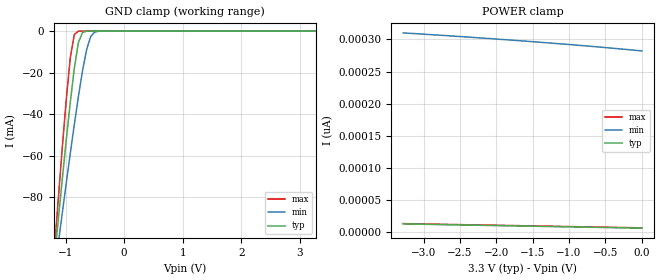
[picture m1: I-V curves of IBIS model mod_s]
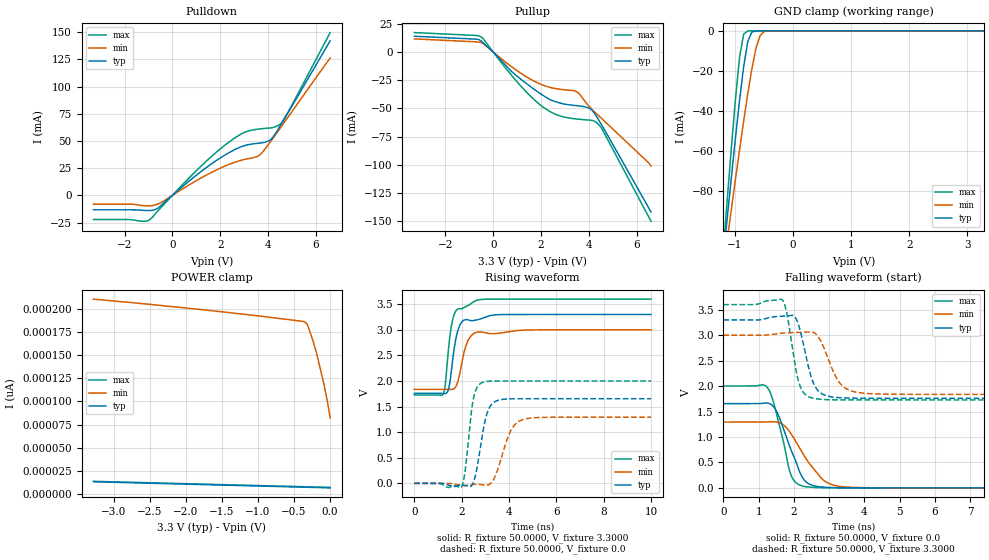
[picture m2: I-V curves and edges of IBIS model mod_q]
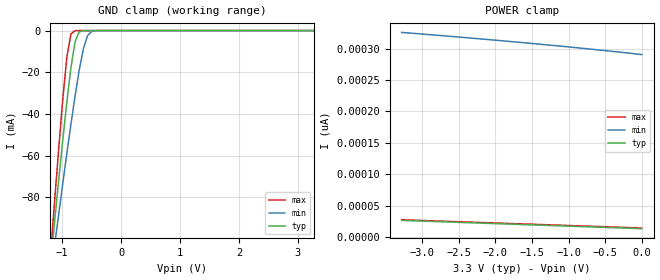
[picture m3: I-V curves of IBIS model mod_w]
| IBIS (I/O, Buffer, Information, Specification) Model, officially
| electronic behavioral standard for Buffer structures of digital pins.
[IBIS ver]  4.0
[File name] m95m02e-a125_3v3_tssop08.ibs
[File Rev]  1.0
[Date]   12 March 2025
[Source]   CAD & Design Services (Catania) - STMicroelectronics
[Notes]
   (Note1)  This IBIS model includes TSSOP8 Package parasitic data
   (Note2)  This IBIS model considers: VCC=3.30(TYP), 3.00(MIN), 3.60(MAX)
   (Note3)  This IBIS model has some Notes about the non-monotonicity
   of the I-V curves, but they are not indicative of problems
   inside the model;
[Disclaimer]
   Customers are solely responsible for all aspects of their
   own product designs or applications using this IBIS Model.
   STMicroelectronics assumes no liability for Custmer Designs
   and applications associated to this IBIS Model.
   In the use of this IBIS Model Customer shall not modify,
   disassemble, alter this Model in whole or in part.
   If Customers do not accept these terms, the IBIS Model
   may not be used. For any problems or modifications please
   contact STMicroelectronics (www.st.com).
[Copyright] (c) 2025 STMicroelectronics
|   Component M95M02E
[Component] M95M02E
[Manufacturer] STMicroelectronics
[Package]
| variable   typ   min   max
R_pkg   0.0   0.0   0.0
L_pkg   0.0H   0.0H   0.0H
C_pkg   0.0F   0.0F   0.0F
[Pin]  signal_name   model_name   R_pin   L_pin   C_pin
1   SN   mod_s   0.0   0.0   0.0
2   Q   mod_q   0.0   0.0   0.0
3   WN   mod_w   0.0   0.0   0.0
4   GND   GND   0.0   0.0   0.0
5   D   mod_d   0.0   0.0   0.0
6   C   mod_c   0.0   0.0   0.0
7   H   mod_h   0.0   0.0   0.0
8   VCC   POWER   0.0   0.0   0.0
[Package Model]  182696_TSSOP8
[Define Package Model]  182696_TSSOP8
[Manufacturer]  STMicroelectronics
[OEM]  STMicroelectronics
[Description]  8 pin TSSOP package
[Number Of Pins]  8
[Pin Numbers]
|Pin Num   Terminal Name
1   | net1
2   | net2
3   | net3
4   | net4_GND
5   | net5
6   | net6
7   | net7
8   | net8_VDD
[Model Data]
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[End Model Data]
[End Package Model]
| Models and submodels in the file (6): mod_s (Input), mod_q (I/O), mod_w (Input), mod_d (Input), mod_c (Input), mod_h (Input)
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|   Model mod_s
[Model]   mod_s
Model_type Input
Vinl   =   0.990V
Vinh   =   2.310V
C_comp   3.207pF   2.940pF   3.586pF
[Temperature Range]  25.0000   0.1250k   -40.0000
[Voltage Range]   3.3000V   3.0000V   3.6000V
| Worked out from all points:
|   GND clamp passes 1 mA (typ) near -0.72 V on its own axis
[GND_clamp]
|Voltage   I(typ)   I(min)   I(max)
-3.3V     -758.5mA   -596.9mA   -944.4mA
-1.2V     -113.1mA   -119mA     -109.3mA
-1.13V    -92.65mA   -103.7mA   -83.15mA
-1.06V    -72.59mA   -88.63mA   -57.71mA
-920mV    -34.54mA   -59.15mA   -13.02mA
-850mV    -17.85mA   -44.98mA   -1.616mA
-780mV    -5.439mA   -31.48mA   -60.01uA
-710mV    -645.3uA   -19.12mA   -1.855uA
-640mV    -45.58uA   -8.894mA   -57.01nA
-570mV    -3.005uA   -2.55mA    -1.764nA
-500mV    -197.3nA   -431.8uA   -57.18pA
3.28V     6.672pA    285.1pA    6.56pA
[POWER_clamp]
|Voltage   I(typ)   I(min)   I(max)
-3.28V    13.31pA    310.2pA    13.76pA
-2.8V     12.35pA    306.8pA    12.8pA
-2.32V    11.38pA    303.2pA    11.84pA
-1.84V    10.42pA    299.4pA    10.88pA
-1.48V    9.692pA    296.4pA    10.16pA
-1.08V    8.887pA    292.9pA    9.36pA
-600mV    7.921pA    288.4pA    8.4pA
0V        6.712pA    282.2pA    7.2pA
|   Model mod_q
[Model]   mod_q
Model_type I/O
Polarity   Non-Inverting
Enable   Active-Low
Vinl   =   0.990V
Vinh   =   2.310V
Vmeas  =   1.650V
Cref   =   30pF
C_comp   3.856pF   3.517pF   4.038pF
[Temperature Range]  25.0000   0.1250k   -40.0000
[Voltage Range]   3.3000V   3.0000V   3.6000V
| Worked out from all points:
|   slope of the pulldown table from 0 to 0.495 V, typ, clamps not added: 52.8 ohm
|   slope of the pullup table from 0 to 0.495 V, typ, clamps not added: 44.4 ohm
|   GND clamp passes 1 mA (typ) near -0.72 V on its own axis
|   rising waveform, R_fixture 50.0000, V_fixture 3.3000: 20-80 % time 313ps typ, 363ps min, 292ps max; typ from 1.76 V to 3.3 V
|   rising waveform, R_fixture 50.0000, V_fixture 0.0: 20-80 % time 384ps typ, 564ps min, 286ps max; typ from 0 V to 1.65 V
|   falling waveform, R_fixture 50.0000, V_fixture 0.0: 20-80 % time 532ps typ, 747ps min, 399ps max; typ from 1.65 V to 0 V
|   falling waveform, R_fixture 50.0000, V_fixture 3.3000: 20-80 % time 334ps typ, 450ps min, 274ps max; typ from 3.3 V to 1.76 V
[Pulldown]
|Voltage   I(typ)   I(min)   I(max)
-3.3V     -13.24mA   -8.114mA   -22.15mA
-1.7V     -13.27mA   -8.123mA   -22.33mA
-1V       -13.97mA   -9.639mA   -23.14mA
-600mV    -11.76mA   -7.819mA   -14.18mA
1V        18.45mA    13.49mA    22.6mA
2.3V      38.37mA    27.82mA    47.83mA
3V        45.61mA    32.94mA    57.72mA
3.6V      47.89mA    36.28mA    60.9mA
4.1V      50.97mA    49.13mA    61.95mA
4.4V      59.9mA     58.29mA    63.97mA
4.6V      67.1mA     64.47mA    67.59mA
6.6V      142mA      126.3mA    149.6mA
[Pullup]
|Voltage   I(typ)   I(min)   I(max)
-3.3V     13.98mA    11.62mA    17.25mA
-800mV    11.56mA    9.122mA    14.78mA
-500mV    9.702mA    8.372mA    13.36mA
1V        -21.45mA   -16.6mA    -26.51mA
2V        -37.34mA   -28.72mA   -47.47mA
2.4V      -42.63mA   -31.51mA   -53.14mA
2.7V      -44.71mA   -32.77mA   -56.02mA
3.5V      -47.66mA   -35.36mA   -59.48mA
4.1V      -50.97mA   -50.32mA   -60.58mA
4.3V      -56.47mA   -54.32mA   -62.25mA
4.5V      -63.47mA   -58.32mA   -66.55mA
6.6V      -142mA     -101.1mA   -150.2mA
[GND_clamp]
|Voltage   I(typ)   I(min)   I(max)
-3.3V     -758.5mA   -596.9mA   -944.4mA
-1.2V     -113.1mA   -119mA     -109.3mA
-1.13V    -92.65mA   -103.7mA   -83.15mA
-1.06V    -72.59mA   -88.63mA   -57.71mA
-920mV    -34.54mA   -59.15mA   -13.02mA
-850mV    -17.85mA   -44.98mA   -1.616mA
-780mV    -5.439mA   -31.48mA   -60.01uA
-710mV    -645.3uA   -19.12mA   -1.855uA
-640mV    -45.58uA   -8.894mA   -57.01nA
-570mV    -3.005uA   -2.55mA    -1.764nA
-500mV    -197.3nA   -431.8uA   -57.18pA
3.28V     6.672pA    285.1pA    6.56pA
[POWER_clamp]
|Voltage   I(typ)   I(min)   I(max)
-3.28V    13.31pA    210.2pA    13.76pA
-1.84V    10.42pA    199.4pA    10.88pA
-360mV    7.438pA    186pA      7.92pA
-320mV    7.357pA    183.5pA    7.84pA
-280mV    7.277pA    175.1pA    7.76pA
-240mV    7.196pA    165.7pA    7.68pA
-200mV    7.115pA    155.3pA    7.6pA
-160mV    7.035pA    142.9pA    7.52pA
-80mV     6.874pA    116pA      7.36pA
-40mV     6.793pA    100.6pA    7.28pA
0V        6.712pA    82.2pA     7.2pA
[Ramp]
| variable   typ   min   max
dV/dt_r  0.9925/0.4859n   0.7756/0.5969n   1.2010/0.4290n
dV/dt_f  0.9244/0.3935n   0.7190/0.4420n   1.1022/0.3693n
R_load = 50.0000
[Rising Waveform]
R_fixture= 50.0000
V_fixture= 3.3000
V_fixture_min= 3.0000
V_fixture_max= 3.6000
|time   V(typ)   V(min)   V(max)
0s        1.759V     1.837V     1.727V
1.22ns    1.757V     1.837V     1.74V
1.32ns    1.756V     1.837V     1.981V
1.46ns    1.867V     1.835V     2.697V
1.68ns    2.619V     1.852V     3.293V
1.84ns    2.985V     1.99V      3.407V
2ns       3.148V     2.334V     3.412V
2.26ns    3.197V     2.781V     3.473V
2.62ns    3.192V     2.95V      3.574V
10ns      3.3V       3V         3.6V
[Rising Waveform]
R_fixture= 50.0000
V_fixture= 0.0
V_fixture_min= 0.0
V_fixture_max= 0.0
|time   V(typ)   V(min)   V(max)
0s        1.226nV    2.702uV    165.9pV
1.99ns    -32.12mV   -41.69mV   -73.76mV
2.15ns    -39.3mV    -45.86mV   251.2mV
2.49ns    13.5mV     -21.32mV   1.639V
2.87ns    929.3mV    -27.57mV   1.97V
3.09ns    1.39V      -33.66mV   1.993V
3.33ns    1.573V     62.1mV     1.999V
4.07ns    1.651V     1.026V     2.001V
4.55ns    1.654V     1.24V      2.001V
10ns      1.654V     1.292V     2.001V
[Falling Waveform]
R_fixture= 50.0000
V_fixture= 0.0
V_fixture_min= 0.0
V_fixture_max= 0.0
|time   V(typ)   V(min)   V(max)
0s        1.654V     1.292V     2.001V
1.26ns    1.665V     1.296V     1.96V
1.38ns    1.625V     1.299V     1.779V
1.52ns    1.49V      1.292V     1.419V
1.9ns     779.2mV    1.083V     286.1mV
2.22ns    230.8mV    711.8mV    41mV
2.42ns    79.58mV    496.7mV    15.47mV
2.82ns    14.53mV    162.6mV    2.518mV
3.3ns     2.422mV    29.29mV    316.4uV
10ns      36.46nV    2.826uV    22.17nV
[Falling Waveform]
R_fixture= 50.0000
V_fixture= 3.3000
V_fixture_min= 3.0000
V_fixture_max= 3.6000
|time   V(typ)   V(min)   V(max)
0s        3.3V       3V         3.6V
1.69ns    3.371V     3.042V     3.68V
1.81ns    3.377V     3.047V     3.393V
2.01ns    3.372V     3.051V     2.507V
2.13ns    3.206V     3.052V     2.092V
2.51ns    2.137V     3.062V     1.766V
2.77ns    1.859V     2.872V     1.739V
3.27ns    1.772V     2.087V     1.728V
3.69ns    1.762V     1.891V     1.727V
10ns      1.759V     1.837V     1.727V
|   Model mod_w
[Model]   mod_w
Model_type Input
Vinl   =   0.990V
Vinh   =   2.310V
C_comp   3.207pF   2.940pF   3.586pF
[Temperature Range]  25.0000   0.1250k   -40.0000
[Voltage Range]   3.3000V   3.0000V   3.6000V
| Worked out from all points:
|   GND clamp passes 1 mA (typ) near -0.72 V on its own axis
[GND_clamp]
|Voltage   I(typ)   I(min)   I(max)
-3.3V     -758.5mA   -596.9mA   -944.4mA
-1.2V     -113.1mA   -119mA     -109.3mA
-1.13V    -92.65mA   -103.7mA   -83.15mA
-1.06V    -72.6mA    -88.63mA   -57.71mA
-920mV    -34.55mA   -59.15mA   -13.02mA
-850mV    -17.86mA   -44.98mA   -1.621mA
-780mV    -5.442mA   -31.48mA   -62.39uA
-710mV    -648.3uA   -19.12mA   -2.115uA
-640mV    -46.41uA   -8.897mA   -66.31nA
-570mV    -3.089uA   -2.553mA   -2.053nA
-500mV    -203.1nA   -433.1uA   -67.98pA
3.28V     13.28pA    294pA      13.12pA
[POWER_clamp]
|Voltage   I(typ)   I(min)   I(max)
-3.28V    26.53pA    325.7pA    27.52pA
-2.6V     23.8pA     319.3pA    24.8pA
-1.88V    20.91pA    312.1pA    21.92pA
-1.36V    18.83pA    306.6pA    19.84pA
-920mV    17.06pA    301.7pA    18.08pA
-520mV    15.45pA    297pA      16.48pA
0V        13.37pA    290.4pA    14.4pA
